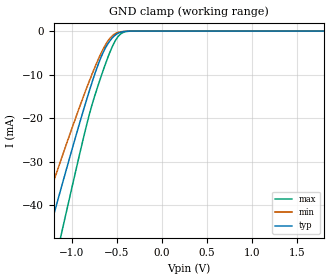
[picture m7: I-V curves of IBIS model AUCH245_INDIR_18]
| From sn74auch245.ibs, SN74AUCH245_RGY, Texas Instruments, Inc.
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[Model]   AUCH245_INDIR_18
Model_type  Input
Vinl=0.5775
Vinh=1.2675
| variable   typ   min   max
C_comp   2.53pF   2.06pF   2.95pF
[Temperature Range]   40   100   -40
| Ambient temperature   25   85   -40
[Voltage range]   1.8   1.65   1.95
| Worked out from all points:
|   GND clamp passes 1 mA (typ) near -0.52 V on its own axis
[GND Clamp]
| AUCH245_INDIR_18
|   Voltage   I(typ)   I(min)   I(max)
-3.6V     -229.3mA   -192.6mA   -273mA
-1.425V   -59.27mA   -48.46mA   -74.95mA
-1.375V   -55.44mA   -45.31mA   -70.36mA
-1.28V    -48.21mA   -39.37mA   -61.64mA
-1.235V   -44.81mA   -36.59mA   -57.52mA
-1.12V    -36.19mA   -29.57mA   -46.99mA
-1.085V   -33.6mA    -27.46mA   -43.79mA
-815mV    -14.38mA   -11.99mA   -19.92mA
-695mV    -7.027mA   -5.991mA   -11.68mA
-550mV    -1.561mA   -1.085mA   -3.576mA
-450mV    -220uA     -142.1uA   -557.1uA
1.8V      305pA      941.6pA    47.06pA
